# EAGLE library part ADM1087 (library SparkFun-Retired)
Power supply sequencer
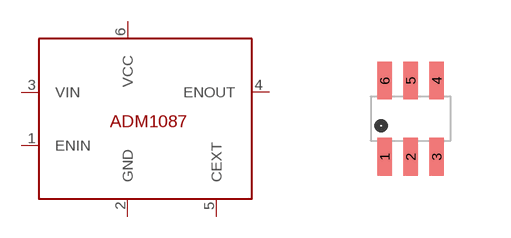
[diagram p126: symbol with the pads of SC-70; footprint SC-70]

Designator prefix -

## ADM1087SC-70  [SC-70]
1  ENIN
2  GND
3  VIN
4  ENOUT
5  CEXT
6  VCC

## Footprint SC-70 (pad centres in mm)
smd 0.36 x 0.95: 1 -0.65,-0.95; 2 0,-0.95; 3 0.65,-0.95; 4 0.65,0.95; 5 0,0.95; 6 -0.65,0.95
